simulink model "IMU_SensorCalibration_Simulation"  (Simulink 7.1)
settings: Solver=FixedStepDiscrete  StartTime=0.0  StopTime=16  FixedStep=.001  RelTol=1e-3
PreLoadFcn:
  | Script_Kalman
undefined symbols (not defined in the file or in its folder): DiscIntNeverNeededParam, float
libraries: simulink x8

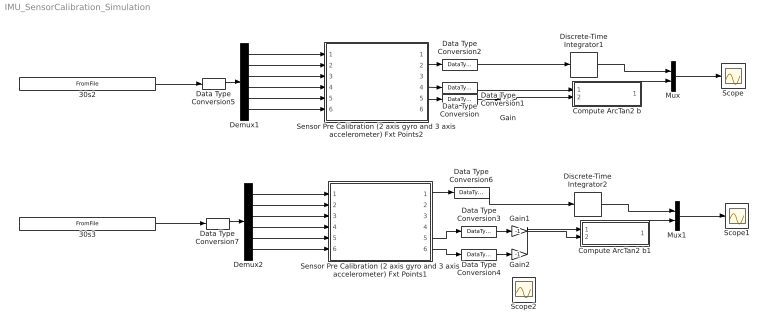
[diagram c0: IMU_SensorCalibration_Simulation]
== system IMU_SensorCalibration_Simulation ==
  30s2 : FromFile  FileName=Pitch_Up_Calibration.mat  SampleTime=.001
  30s3 : FromFile  FileName=Roll_Right_Calibration.mat  SampleTime=.001
  Compute ArcTan2 b : Subsystem
  Compute ArcTan2 b1 : Subsystem
  Data Type Conversion{,1..4,6} (6 alike) : DataTypeConversion  OutDataType=sfix(16)  OutScaling=2^0
  Data Type Conversion5 : DataTypeConversion  OutDataTypeMode=int16  OutDataType=sfix(16)  OutScaling=2^0  OutDataTypeStr=int16
  Data Type Conversion7 : DataTypeConversion  OutDataTypeMode=int16  OutDataType=sfix(16)  OutScaling=2^0  OutDataTypeStr=int16
  Demux1 : Demux  Outputs=6
  Demux2 : Demux  Outputs=6
  Discrete-Time Integrator1 : DiscreteIntegrator  SampleTime=.001  OutDataType=sfix(16)  OutScaling=2^0  ICPrevOutput=DiscIntNeverNeededParam  ICPrevScaledInput=DiscIntNeverNeededParam
  Discrete-Time Integrator2 : DiscreteIntegrator  SampleTime=.001  OutDataType=sfix(16)  OutScaling=2^0  ICPrevOutput=DiscIntNeverNeededParam  ICPrevScaledInput=DiscIntNeverNeededParam
  Gain : Gain  Gain=-1  ParameterDataType=sfix(16)  ParameterScaling=2^0  OutDataType=sfix(16)  OutScaling=2^0
  Gain1 : Gain  Gain=-1  ParameterDataType=sfix(16)  ParameterScaling=2^0  OutDataType=sfix(16)  OutScaling=2^0
  Gain2 : Gain  Gain=-1  ParameterDataType=sfix(16)  ParameterScaling=2^0  OutDataType=sfix(16)  OutScaling=2^0
  Mux : Mux  Inputs=2
  Mux1 : Mux  Inputs=2
  Scope : Scope
  Scope1 : Scope
  Scope2 : Scope  NumInputPorts=3
  Sensor Pre Calibration (2 axis gyro and 3 axis accelerometer) Fxt Points1 : Subsystem
  Sensor Pre Calibration (2 axis gyro and 3 axis accelerometer) Fxt Points2 : Subsystem
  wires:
  Data Type Conversion5/1 -> Demux1/1
  30s2/1 -> Data Type Conversion5/1
  Demux1/1 -> Sensor Pre Calibration (2 axis gyro and 3 axis accelerometer) Fxt Points2/1(Gyro Y)
  Demux1/2 -> Sensor Pre Calibration (2 axis gyro and 3 axis accelerometer) Fxt Points2/2(Accel y)
  Demux1/3 -> Sensor Pre Calibration (2 axis gyro and 3 axis accelerometer) Fxt Points2/3(Accel z)
  Demux1/4 -> Sensor Pre Calibration (2 axis gyro and 3 axis accelerometer) Fxt Points2/4(Gyro X)
  Demux1/5 -> Sensor Pre Calibration (2 axis gyro and 3 axis accelerometer) Fxt Points2/5(Accel x)
  Demux1/6 -> Sensor Pre Calibration (2 axis gyro and 3 axis accelerometer) Fxt Points2/6(Gyro z)
  Sensor Pre Calibration (2 axis gyro and 3 axis accelerometer) Fxt Points2/4(unbiased Accel Y) -> Data Type Conversion/1
  Sensor Pre Calibration (2 axis gyro and 3 axis accelerometer) Fxt Points2/5(unbiased Accel X) -> Data Type Conversion1/1
  Sensor Pre Calibration (2 axis gyro and 3 axis accelerometer) Fxt Points2/2(Gyro X (degree/s)) -> Data Type Conversion2/1
  Discrete-Time Integrator1/1 -> Mux/1
  Compute ArcTan2 b/1(Degree) -> Mux/2
  Mux/1 -> Scope/1
  Data Type Conversion2/1 -> Discrete-Time Integrator1/1
  Data Type Conversion1/1 -> Gain/1
  Gain/1 -> Compute ArcTan2 b/2(Force 2)
  Data Type Conversion/1 -> Compute ArcTan2 b/1(Force 1)
  Data Type Conversion7/1 -> Demux2/1
  30s3/1 -> Data Type Conversion7/1
  Demux2/1 -> Sensor Pre Calibration (2 axis gyro and 3 axis accelerometer) Fxt Points1/1(Gyro Y)
  Demux2/2 -> Sensor Pre Calibration (2 axis gyro and 3 axis accelerometer) Fxt Points1/2(Accel y)
  Demux2/3 -> Sensor Pre Calibration (2 axis gyro and 3 axis accelerometer) Fxt Points1/3(Accel z)
  Demux2/4 -> Sensor Pre Calibration (2 axis gyro and 3 axis accelerometer) Fxt Points1/4(Gyro X)
  Demux2/5 -> Sensor Pre Calibration (2 axis gyro and 3 axis accelerometer) Fxt Points1/5(Accel x)
  Demux2/6 -> Sensor Pre Calibration (2 axis gyro and 3 axis accelerometer) Fxt Points1/6(Gyro z)
  Discrete-Time Integrator2/1 -> Mux1/1
  Compute ArcTan2 b1/1(Degree) -> Mux1/2
  Mux1/1 -> Scope1/1
  Data Type Conversion6/1 -> Discrete-Time Integrator2/1
  Sensor Pre Calibration (2 axis gyro and 3 axis accelerometer) Fxt Points1/1(Gyro Y (degree/s)) -> Data Type Conversion6/1
  Sensor Pre Calibration (2 axis gyro and 3 axis accelerometer) Fxt Points1/6(unbiased Accel Z) -> Data Type Conversion4/1
  Sensor Pre Calibration (2 axis gyro and 3 axis accelerometer) Fxt Points1/5(unbiased Accel X) -> Data Type Conversion3/1
  Data Type Conversion4/1 -> Gain2/1
  Data Type Conversion3/1 -> Gain1/1
  Gain1/1 -> Compute ArcTan2 b1/2(Force 2)
  Gain2/1 -> Compute ArcTan2 b1/1(Force 1)

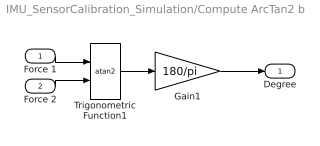
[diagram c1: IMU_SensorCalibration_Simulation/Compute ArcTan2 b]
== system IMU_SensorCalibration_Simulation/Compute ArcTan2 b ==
  Force 1 : Inport
  Force 2 : Inport  Port=2
  Gain1 : Gain  Gain=180/pi  ParameterDataType=sfix(16)  ParameterScaling=2^0  OutDataTypeMode=Specify via dialog  OutDataType=float('double')  OutDataTypeStr=float('double')
  Trigonometric Function1 : Trigonometry  Operator=atan2  OutputSignalType=real
  Degree : Outport
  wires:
  Trigonometric Function1/1 -> Gain1/1
  Gain1/1 -> Degree/1
  Force 1/1 -> Trigonometric Function1/1
  Force 2/1 -> Trigonometric Function1/2

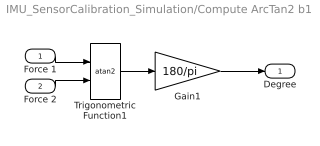
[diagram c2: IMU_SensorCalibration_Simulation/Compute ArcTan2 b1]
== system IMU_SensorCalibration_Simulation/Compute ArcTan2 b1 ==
  Force 1 : Inport
  Force 2 : Inport  Port=2
  Gain1 : Gain  Gain=180/pi  ParameterDataType=sfix(16)  ParameterScaling=2^0  OutDataTypeMode=Specify via dialog  OutDataType=float('double')  OutDataTypeStr=float('double')
  Trigonometric Function1 : Trigonometry  Operator=atan2  OutputSignalType=real
  Degree : Outport
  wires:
  Force 2/1 -> Trigonometric Function1/2
  Force 1/1 -> Trigonometric Function1/1
  Gain1/1 -> Degree/1
  Trigonometric Function1/1 -> Gain1/1

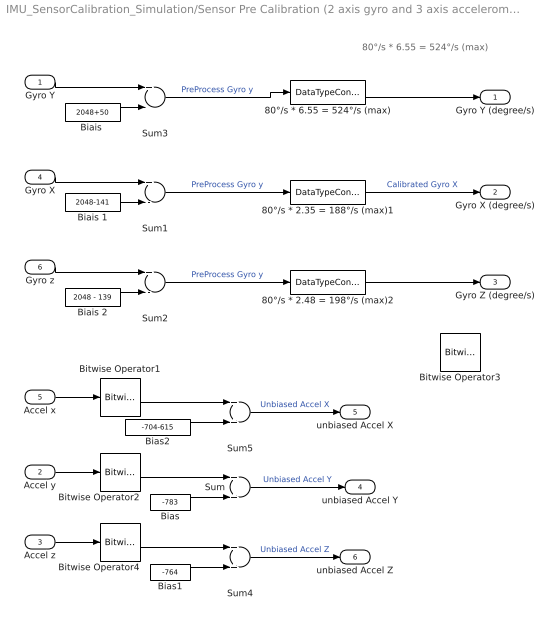
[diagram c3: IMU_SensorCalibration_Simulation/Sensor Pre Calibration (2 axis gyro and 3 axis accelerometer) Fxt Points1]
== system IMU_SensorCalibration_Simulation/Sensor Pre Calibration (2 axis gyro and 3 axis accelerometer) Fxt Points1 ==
  note: 80°/s * 6.55 = 524°/s (max)
  Gyro Y : Inport
  Accel y : Inport  Port=2
  Accel z : Inport  Port=3
  Gyro X : Inport  Port=4
  Accel x : Inport  Port=5
  Gyro z : Inport  Port=6
  80°/s * 2.35 = 188°/s (max)1 : DataTypeConversion  OutDataTypeMode=Specify via dialog  OutDataType=fixdt(1,16,80/2048*2.49,0)  OutDataTypeStr=fixdt(1,16,80/2048*2.49,0)  ConvertRealWorld=Stored Integer (SI)
  80°/s * 2.48 = 198°/s (max)2 : DataTypeConversion  OutDataTypeMode=Specify via dialog  OutDataType=fixdt(1,16,80/2048*2.5,0)  OutDataTypeStr=fixdt(1,16,80/2048*2.5,0)  ConvertRealWorld=Stored Integer (SI)
  80°/s * 6.55 = 524°/s (max) : DataTypeConversion  OutDataTypeMode=Specify via dialog  OutDataType=fixdt(1,16,80/2048*4.93,0)  OutDataTypeStr=fixdt(1,16,80/2048*4.93,0)  ConvertRealWorld=Stored Integer (SI)
  "Biais " : Constant  Value=2048+50  OutDataType=sfix(16)  OutScaling=2^0  OutDataTypeStr=Inherit: Inherit via back propagation
  Biais 1 : Constant  Value=2048-141  OutDataType=sfix(16)  OutScaling=2^0  OutDataTypeStr=Inherit: Inherit via back propagation
  Biais 2 : Constant  Value=2048 - 139  OutDataType=sfix(16)  OutScaling=2^0  OutDataTypeStr=Inherit: Inherit via back propagation
  Bias : Constant  Value=-783  OutDataType=sfix(16)  OutScaling=2^0  OutDataTypeStr=Inherit: Inherit via back propagation
  Bias1 : Constant  Value=-764  OutDataType=sfix(16)  OutScaling=2^0  OutDataTypeStr=Inherit: Inherit via back propagation
  Bias2 : Constant  Value=-704-615  OutDataType=sfix(16)  OutScaling=2^0  OutDataTypeStr=Inherit: Inherit via back propagation
  Bitwise Operator{1..4} (4 alike) : simulink/Logic and Bit Operations/Bitwise Operator  logicop=AND  UseBitMask=on  BitMask=4095  BitMaskRealWorld=Stored Integer
  Sum : Sum  AccumDataTypeStr=int16  OutDataTypeMode=int16  OutDataType=sfix(16)  OutScaling=2^0  OutDataTypeStr=int16
  Sum1 : Sum  Inputs=+-  AccumDataTypeStr=int16  OutDataTypeMode=int16  OutDataType=sfix(16)  OutScaling=2^0  OutDataTypeStr=int16
  Sum2 : Sum  Inputs=+-  AccumDataTypeStr=int16  OutDataTypeMode=int16  OutDataType=sfix(16)  OutScaling=2^0  OutDataTypeStr=int16
  Sum3 : Sum  Inputs=+-  AccumDataTypeStr=int16  OutDataTypeMode=int16  OutDataType=sfix(16)  OutScaling=2^0  OutDataTypeStr=int16
  Sum4 : Sum  AccumDataTypeStr=int16  OutDataTypeMode=int16  OutDataType=sfix(16)  OutScaling=2^0  OutDataTypeStr=int16
  Sum5 : Sum  AccumDataTypeStr=int16  OutDataTypeMode=int16  OutDataType=sfix(16)  OutScaling=2^0  OutDataTypeStr=int16
  Gyro Y (degree/s) : Outport
  Gyro X (degree/s) : Outport  Port=2
  Gyro Z (degree/s) : Outport  Port=3
  unbiased Accel Y : Outport  Port=4
  unbiased Accel X : Outport  Port=5
  unbiased Accel Z : Outport  Port=6
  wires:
  Gyro X/1 -> Sum1/1
  Biais 1/1 -> Sum1/2
  Gyro Y/1 -> Sum3/1
  "Biais "/1 -> Sum3/2
  Gyro z/1 -> Sum2/1
  Biais 2/1 -> Sum2/2
  Accel z/1 -> Bitwise Operator4/1
  Accel y/1 -> Bitwise Operator2/1
  Sum3/1 -> 80°/s * 6.55 = 524°/s (max)/1  "PreProcess Gyro y"
  Sum2/1 -> 80°/s * 2.48 = 198°/s (max)2/1  "PreProcess Gyro y"
  Bias/1 -> Sum/2
  Bias1/1 -> Sum4/2
  Bias2/1 -> Sum5/2
  Sum/1 -> unbiased Accel Y/1  "Unbiased Accel Y"
  Sum4/1 -> unbiased Accel Z/1  "Unbiased Accel Z"
  Sum5/1 -> unbiased Accel X/1  "Unbiased Accel X"
  80°/s * 6.55 = 524°/s (max)/1 -> Gyro Y (degree/s)/1
  80°/s * 2.35 = 188°/s (max)1/1 -> Gyro X (degree/s)/1  "Calibrated Gyro X"
  80°/s * 2.48 = 198°/s (max)2/1 -> Gyro Z (degree/s)/1
  Sum1/1 -> 80°/s * 2.35 = 188°/s (max)1/1  "PreProcess Gyro y"
  Accel x/1 -> Bitwise Operator1/1
  Bitwise Operator1/1 -> Sum5/1
  Bitwise Operator2/1 -> Sum/1
  Bitwise Operator4/1 -> Sum4/1

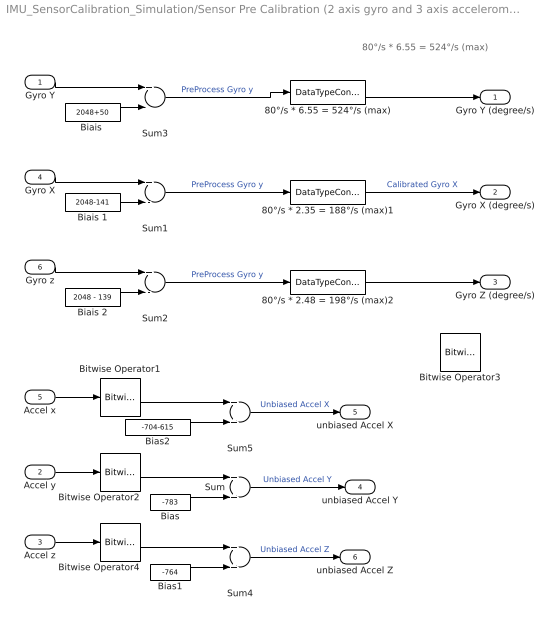
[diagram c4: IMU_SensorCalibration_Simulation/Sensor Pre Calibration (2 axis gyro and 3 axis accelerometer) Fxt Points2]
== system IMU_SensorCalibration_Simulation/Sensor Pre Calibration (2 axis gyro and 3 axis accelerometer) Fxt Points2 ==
  note: 80°/s * 6.55 = 524°/s (max)
  Gyro Y : Inport
  Accel y : Inport  Port=2
  Accel z : Inport  Port=3
  Gyro X : Inport  Port=4
  Accel x : Inport  Port=5
  Gyro z : Inport  Port=6
  80°/s * 2.35 = 188°/s (max)1 : DataTypeConversion  OutDataTypeMode=Specify via dialog  OutDataType=fixdt(1,16,80/2048*2.49,0)  OutDataTypeStr=fixdt(1,16,80/2048*2.49,0)  ConvertRealWorld=Stored Integer (SI)
  80°/s * 2.48 = 198°/s (max)2 : DataTypeConversion  OutDataTypeMode=Specify via dialog  OutDataType=fixdt(1,16,80/2048*2.5,0)  OutDataTypeStr=fixdt(1,16,80/2048*2.5,0)  ConvertRealWorld=Stored Integer (SI)
  80°/s * 6.55 = 524°/s (max) : DataTypeConversion  OutDataTypeMode=Specify via dialog  OutDataType=fixdt(1,16,80/2048*4.93,0)  OutDataTypeStr=fixdt(1,16,80/2048*4.93,0)  ConvertRealWorld=Stored Integer (SI)
  "Biais " : Constant  Value=2048+50  OutDataType=sfix(16)  OutScaling=2^0  OutDataTypeStr=Inherit: Inherit via back propagation
  Biais 1 : Constant  Value=2048-141  OutDataType=sfix(16)  OutScaling=2^0  OutDataTypeStr=Inherit: Inherit via back propagation
  Biais 2 : Constant  Value=2048 - 139  OutDataType=sfix(16)  OutScaling=2^0  OutDataTypeStr=Inherit: Inherit via back propagation
  Bias : Constant  Value=-783  OutDataType=sfix(16)  OutScaling=2^0  OutDataTypeStr=Inherit: Inherit via back propagation
  Bias1 : Constant  Value=-764  OutDataType=sfix(16)  OutScaling=2^0  OutDataTypeStr=Inherit: Inherit via back propagation
  Bias2 : Constant  Value=-704-615  OutDataType=sfix(16)  OutScaling=2^0  OutDataTypeStr=Inherit: Inherit via back propagation
  Bitwise Operator{1..4} (4 alike) : simulink/Logic and Bit Operations/Bitwise Operator  logicop=AND  UseBitMask=on  BitMask=4095  BitMaskRealWorld=Stored Integer
  Sum : Sum  AccumDataTypeStr=int16  OutDataTypeMode=int16  OutDataType=sfix(16)  OutScaling=2^0  OutDataTypeStr=int16
  Sum1 : Sum  Inputs=+-  AccumDataTypeStr=int16  OutDataTypeMode=int16  OutDataType=sfix(16)  OutScaling=2^0  OutDataTypeStr=int16
  Sum2 : Sum  Inputs=+-  AccumDataTypeStr=int16  OutDataTypeMode=int16  OutDataType=sfix(16)  OutScaling=2^0  OutDataTypeStr=int16
  Sum3 : Sum  Inputs=+-  AccumDataTypeStr=int16  OutDataTypeMode=int16  OutDataType=sfix(16)  OutScaling=2^0  OutDataTypeStr=int16
  Sum4 : Sum  AccumDataTypeStr=int16  OutDataTypeMode=int16  OutDataType=sfix(16)  OutScaling=2^0  OutDataTypeStr=int16
  Sum5 : Sum  AccumDataTypeStr=int16  OutDataTypeMode=int16  OutDataType=sfix(16)  OutScaling=2^0  OutDataTypeStr=int16
  Gyro Y (degree/s) : Outport
  Gyro X (degree/s) : Outport  Port=2
  Gyro Z (degree/s) : Outport  Port=3
  unbiased Accel Y : Outport  Port=4
  unbiased Accel X : Outport  Port=5
  unbiased Accel Z : Outport  Port=6
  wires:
  Bitwise Operator4/1 -> Sum4/1
  Bitwise Operator2/1 -> Sum/1
  Bitwise Operator1/1 -> Sum5/1
  Accel x/1 -> Bitwise Operator1/1
  Sum1/1 -> 80°/s * 2.35 = 188°/s (max)1/1  "PreProcess Gyro y"
  80°/s * 2.48 = 198°/s (max)2/1 -> Gyro Z (degree/s)/1
  80°/s * 2.35 = 188°/s (max)1/1 -> Gyro X (degree/s)/1  "Calibrated Gyro X"
  80°/s * 6.55 = 524°/s (max)/1 -> Gyro Y (degree/s)/1
  Sum5/1 -> unbiased Accel X/1  "Unbiased Accel X"
  Sum4/1 -> unbiased Accel Z/1  "Unbiased Accel Z"
  Sum/1 -> unbiased Accel Y/1  "Unbiased Accel Y"
  Bias2/1 -> Sum5/2
  Bias1/1 -> Sum4/2
  Bias/1 -> Sum/2
  Sum2/1 -> 80°/s * 2.48 = 198°/s (max)2/1  "PreProcess Gyro y"
  Sum3/1 -> 80°/s * 6.55 = 524°/s (max)/1  "PreProcess Gyro y"
  Accel y/1 -> Bitwise Operator2/1
  Accel z/1 -> Bitwise Operator4/1
  Biais 2/1 -> Sum2/2
  Gyro z/1 -> Sum2/1
  "Biais "/1 -> Sum3/2
  Gyro Y/1 -> Sum3/1
  Biais 1/1 -> Sum1/2
  Gyro X/1 -> Sum1/1
